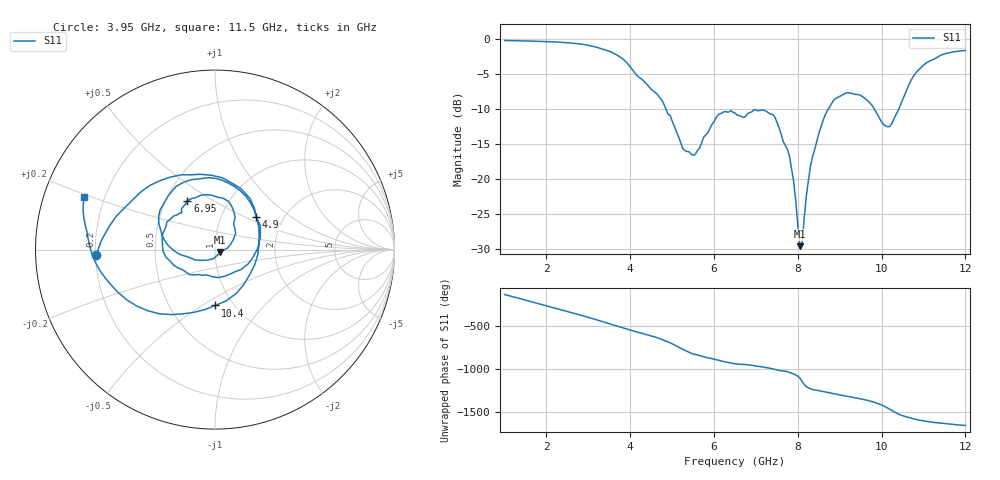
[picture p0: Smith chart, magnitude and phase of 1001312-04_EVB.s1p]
! 1/26/2023 7:03:41 AM
! D:\1001312-04WITHMATCHING.S1P
! CHANNEL.1
! TR.MEASUREMENT
! CORRECTED.DATA
! RF.CORRECTION: ONE.PORT.CAL.PORT[1]
! AVERAGING.OFF
! IF.BANDWIDTH: 1KHZ
! SWEEPTYPE:  FREQ.SWEEP(Linear)
! Reference Plane Port Info
! PORT:  PORT1
! DISTANCE:  6.574 mm
! TIME:  21.9357 ps
! PHASE.OFFSET:  0 °
! LOSS:  0  dB
! REF.LOSS:  0  dB
! REF.FREQ:  1 GHz
! Power Info
! POWER:  -10  dBm
! EFF.POWER:  -10  dBm
! SOURCE.ATTEN:  0  dB
! TEST.ATTEN:  0  dB
# GHZ S RI R 50.0
! FREQ.GHZ  S11RE  S11IM
!; PortSelection: Port_1
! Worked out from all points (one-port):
!   221 points, 1 GHz to 12 GHz, reference 50 ohm
!   lowest |S11| = -29.6 dB at 8.05 GHz (marker M1), VSWR 1.07, Z = 53 - j1.65 ohm
!   |S11| at or under -10 dB: 4.853 GHz to 8.728 GHz (3.875 GHz wide, 57.1 % of centre); 9.829 GHz to 10.41 GHz (580.5 MHz wide, 5.74 % of centre)
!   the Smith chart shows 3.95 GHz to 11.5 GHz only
!   S11 on the Smith chart (normalised r, x): 3.95 GHz: 0.20, -0.02; 4.9 GHz: 1.46, +0.57; 6.95 GHz: 0.64, +0.39; 10.4 GHz: 0.83, -0.57; 11.5 GHz: 0.12, +0.19
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1  -0.5869 -0.7847
1.3  -0.9453 -0.2361
1.6  -0.875 0.4194
2  -0.1877 0.9441
2.4  0.6375 0.7043
2.8  0.9189 -0.1122
3.2  0.3826 -0.7881
3.45  -0.1535 -0.8172
3.75  -0.623 -0.4118
3.95  -0.6619 -0.0309
4.45  -0.1878 0.4169
4.9  0.229 0.1801
5.15  0.1867 -0.0778
5.55  -0.0518 -0.141
6.1  -0.2898 -0.0089
6.5  -0.2306 0.1874
6.95  -0.1538 0.2728
7.45  0.0765 0.268
7.9  0.0902 0.0341
8.05  0.0293 -0.0156
8.55  -0.2359 -0.000121
9.25  -0.1542 0.3831
9.95  0.2443 0.1214
10.4  0.00177 -0.3114
10.65  -0.3087 -0.358
11.05  -0.6677 -0.0692
11.5  -0.7286 0.2926
12  -0.6017 0.5728
